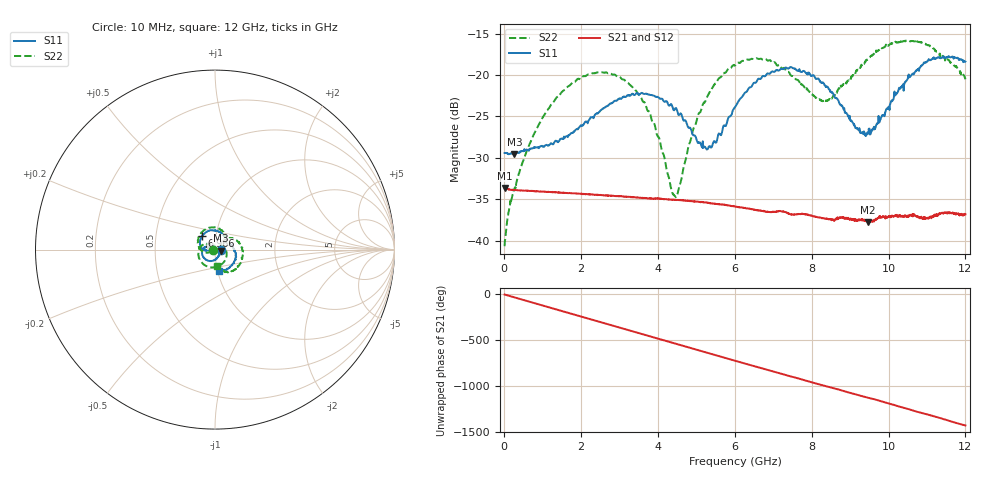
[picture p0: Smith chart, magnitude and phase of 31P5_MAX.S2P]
!Agilent Technologies,E5071C,MY46316741,A.11.02
!Date: Wed Sep 16 11:45:58 2020
!Data & Calibration Information:
!Freq	S11:SOLT2(ON)	S21:SOLT2(ON)	S12:SOLT2(ON)	S22:SOLT2(ON)
!PortZ  Port1:50+j0  Port2:50+j0
!Above PortZ is port z conversion or system Z0 setting when saving the data.
!When reading, reference impedance value at option line is always used.
# Hz S dB R 50
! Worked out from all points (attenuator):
!   1561 points, 10 MHz to 12 GHz, reference 50 ohm
!   highest |S21| = -33.63 dB at 17.69 MHz (marker M1); lowest = -37.8 dB at 9.471 GHz (marker M2)
!   lowest |S11| = -29.6 dB at 263.6 MHz (marker M3), VSWR 1.07, Z = 53.4 - j0.706 ohm
!   |S11| at or under -10 dB: start of sweep to end of sweep
!   |S22| runs from -40.7 to -15.8 dB; largest |S21 - S12| = 0.00055
!   S11 on the Smith chart (normalised r, x): 10 MHz: 1.07, -0.00; 6.966 GHz: 0.86, +0.13; 12 GHz: 1.02, -0.24
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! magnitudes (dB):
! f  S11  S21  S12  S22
! 10 MHz  -29.4  -33.6  -33.6  -40.7
! 17.69 MHz  -29.4  -33.6  -33.7  -40.0
! 263.6 MHz  -29.6  -33.9  -33.9  -33.7
! 609.5 MHz  -29.1  -33.9  -34.0  -28.9
! 1.032 GHz  -28.7  -34.1  -34.1  -24.9
! 2.016 GHz  -26.1  -34.3  -34.4  -20.3
! 3.161 GHz  -22.6  -34.7  -34.7  -20.8
! 3.638 GHz  -22.3  -34.8  -34.9  -23.3
! 4.007 GHz  -22.7  -34.9  -34.9  -27.5
! 4.36 GHz  -23.6  -35.1  -35.0  -34.0
! 4.468 GHz  -24.0  -35.1  -35.1  -34.8
! 4.914 GHz  -27.3  -35.2  -35.3  -26.6
! 5.275 GHz  -29.0  -35.4  -35.4  -22.7
! 6.005 GHz  -23.9  -35.9  -35.9  -18.8
! 6.966 GHz  -19.6  -36.6  -36.6  -18.5
! 8.011 GHz  -20.1  -37.0  -37.0  -22.3
! 8.495 GHz  -22.0  -37.4  -37.4  -22.9
! 9.164 GHz  -26.5  -37.5  -37.4  -19.4
! 9.471 GHz  -27.0  -37.8  -37.7  -18.1
! 10 GHz  -23.8  -37.1  -37.1  -16.4
! 11.02 GHz  -18.3  -37.2  -37.4  -16.4
! 12 GHz  -18.4  -36.8  -36.8  -20.5
